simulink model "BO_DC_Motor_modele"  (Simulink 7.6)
settings: Solver=ode15s  StartTime=0.0  StopTime=100  RelTol=1e-3
StopFcn:
  | load BO_pos_vit.mat
  | delete *.mat
  | plot(x(1,:),x(2,:), x(1,:),x(3,:),x(1,:),x(4,:),'*')
  | grid
  | title('Commande en BO de la vitesse linéaire du Moteur DC')
  | gtext('Commande)')
  | gtext('Vitesse linéaire')
  | xlabel('temps')
libraries: fl_lib x13, nesl_utility x4, elec_lib x1

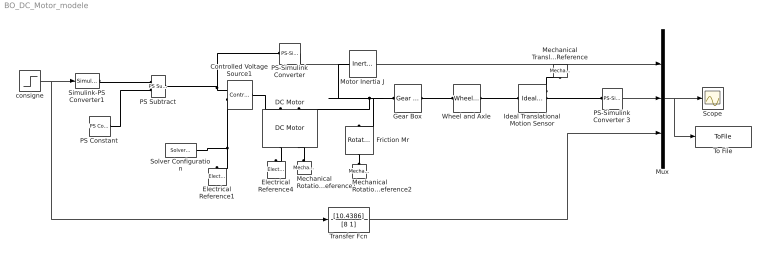
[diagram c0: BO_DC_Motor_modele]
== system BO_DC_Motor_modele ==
  Controlled Voltage Source1 : fl_lib/Electrical/Electrical Sources/Controlled Voltage Source  DialogController=NetworkEngine.DynNeDlgSource  SystemSampleTime=-1  i_Log=off  v_Log=off  LocalVarNames=|current|voltage|power  LocalVarDescs=|Current (A)|Voltage (V)|Power (W)  LocalVarLogging=[0 0 0]
  DC Motor : elec_lib/Actuators & Drivers/Rotational Actuators/DC Motor  DialogController=NetworkEngine.DynNeDlgSource  SystemSampleTime=-1  parameterization=1  Ra=3.9 Ohm  La=1.2e-05 H  emf_or_torque=1  Kv=7.2e-05 V/rpm  Ki=6.876e-04 N*m/A  T_stall=2.4e-04 N*m  w_max=1.91e+04 rpm  w_rated=1.5e+04 rpm  P_rated=0.08 W  V_rated=1.5 V  J=0.01 g*cm^2  lam=1e-08 N*m/(rad/s)  speed0=0 rpm  current_Log=off  voltage_Log=off  power_Log=off  i2r_Log=off  torque_Log=off  speed_Log=off  LocalVarNames=|current|voltage|power|i2r|torque|speed  LocalVarDescs=|Current (A)|Voltage (V)|Power (W)|Electrical losses (W)|Torque (Nm)|Angular speed (rad/s)  LocalVarLogging=[0 0 0 0 0 0]
  Electrical Reference1 : fl_lib/Electrical/Electrical Elements/Electrical Reference  DialogController=NetworkEngine.DynNeDlgSource  SystemSampleTime=-1  i_Log=off  LocalVarNames=|i  LocalVarDescs=|i  LocalVarLogging=[]
  Electrical Reference4 : fl_lib/Electrical/Electrical Elements/Electrical Reference  DialogController=NetworkEngine.DynNeDlgSource  SystemSampleTime=-1  i_Log=off  LocalVarNames=|i  LocalVarDescs=|i  LocalVarLogging=[]
  Friction Mr : fl_lib/Mechanical/Rotational Elements/Rotational Friction  DialogController=NetworkEngine.DynNeDlgSource  SystemSampleTime=-1  brkwy_trq=0.02e-3 N*m  Col_trq=0.02e-3 N*m  visc_coef=0 N*m/(rad/s)  trans_coef=10 s/rad  vel_thr=0.1 rad/s  t_Log=off  w_Log=off  LocalVarNames=|friction_torque|rel_velocity|power  LocalVarDescs=|Friction torque (N*m)|Relative velocity (rad/s)|Power (W)  LocalVarLogging=[0 0 0]
  Gear Box : fl_lib/Mechanical/Mechanisms/Gear Box  DialogController=NetworkEngine.DynNeDlgSource  SystemSampleTime=-1  ratio=5  t_in_Log=off  t_out_Log=off  LocalVarNames=|t_in|t_out  LocalVarDescs=|t_in|t_out  LocalVarLogging=[0 0]
  Ideal Translational Motion Sensor : fl_lib/Mechanical/Mechanical Sensors/Ideal Translational Motion Sensor  DialogController=NetworkEngine.DynNeDlgSource  SystemSampleTime=-1  offset=0 m  v_Log=off  f_Log=off  x_Log=off  LocalVarNames=|v|f|x  LocalVarDescs=|v|f|x  LocalVarLogging=[0 0 0]
  Mechanical Rotational Reference1 : fl_lib/Mechanical/Rotational Elements/Mechanical Rotational Reference  DialogController=NetworkEngine.DynNeDlgSource  SystemSampleTime=-1  t_Log=off  LocalVarNames=|t  LocalVarDescs=|t  LocalVarLogging=[]
  Mechanical Rotational Reference2 : fl_lib/Mechanical/Rotational Elements/Mechanical Rotational Reference  DialogController=NetworkEngine.DynNeDlgSource  SystemSampleTime=-1  t_Log=off  LocalVarNames=|t  LocalVarDescs=|t  LocalVarLogging=[]
  Mechanical Translational Reference : fl_lib/Mechanical/Translational Elements/Mechanical Translational Reference  DialogController=NetworkEngine.DynNeDlgSource  SystemSampleTime=-1  f_Log=off  LocalVarNames=|f  LocalVarDescs=|f  LocalVarLogging=0
  Motor Inertia J : fl_lib/Mechanical/Rotational Elements/Inertia  DialogController=NetworkEngine.DynNeDlgSource  SystemSampleTime=-1  inertia=10 g*cm^2  initial_velocity=0 rad/s  t_Log=off  LocalVarNames=|torque|velocity  LocalVarDescs=|Inertia torque (N*m)|Inertia absolute velocity (rad/s)  LocalVarLogging=[0 0]
  Mux : Mux  Inputs=3
  PS Constant : fl_lib/Physical Signals/Sources/PS Constant  DialogController=NetworkEngine.DynNeDlgSource  SystemSampleTime=-1  constant=0  LocalVarLogging=[]
  PS Subtract : fl_lib/Physical Signals/Functions/PS Subtract  DialogController=NetworkEngine.DynNeDlgSource  SystemSampleTime=-1  LocalVarLogging=[]
  PS-Simulink Converter : nesl_utility/PS-Simulink Converter  DialogController=NetworkEngine.DynNeUtilDlgSource  SystemSampleTime=-1  PhysicalDomain=network_engine_domain  LeftPortType=input  RightPortType=output  SubClassName=ps_output  Unit=1  AffineConversion=off
  PS-Simulink Converter 3 : nesl_utility/PS-Simulink Converter  DialogController=NetworkEngine.DynNeUtilDlgSource  SystemSampleTime=-1  PhysicalDomain=network_engine_domain  LeftPortType=input  RightPortType=output  SubClassName=ps_output  Unit=1  AffineConversion=off
  Scope : Scope
  Simulink-PS Converter1 : nesl_utility/Simulink-PS Converter  DialogController=NetworkEngine.DynNeUtilDlgSource  SystemSampleTime=-1  PhysicalDomain=network_engine_domain  LeftPortType=input  RightPortType=output  SubClassName=ps_input  Unit=1  AffineConversion=off  InputFilterTimeConstant=.001  UdotUserProvided=0
  Solver Configuration : nesl_utility/Solver Configuration  DialogController=NetworkEngine.DynNeUtilDlgSource  SystemSampleTime=-1  PhysicalDomain=network_engine_domain  LeftPortType=input  RightPortType=generic  SubClassName=solver  Accelerate=off  Profile=off  ResidualTolerance=1e-9  MaxNonlinIter=12  MaxModeIter=2  DoFixedCost=off  UseLocalSampling=off  DoDC=off  LinearAlgebra=Full  LocalSolverSampleTime=.001  LocalSolverChoice=NE_BACKWARD_EULER_ADVANCER  UseLocalSolver=off
  To File : ToFile  Filename=BO_pos_vit.mat  MatrixName=x
  Transfer Fcn : TransferFcn  Numerator=[10.4386]  Denominator=[8 1]
  Wheel and Axle : fl_lib/Mechanical/Mechanisms/Wheel and Axle  DialogController=NetworkEngine.DynNeDlgSource  SystemSampleTime=-1  R=0.05 m  or=1  torque_A_Log=off  force_P_Log=off  ang_velocity_Log=off  velocity_Log=off  LocalVarNames=|torque_A|force_P|ang_velocity|velocity  LocalVarDescs=|Axle torque (N*m)|Periphery force (N)|Axle angular velocity (rad/s)|Periphery velocity (m/s)  LocalVarLogging=[0 0 0 0]
  consigne : Step  Time=10  After=0.5  SampleTime=0
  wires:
  Mux/1 -> To File/1, Scope/1
  consigne/1 -> Simulink-PS Converter1/1, Transfer Fcn/1
  PS-Simulink Converter 3/1 -> Mux/2
  PS-Simulink Converter/1 -> Mux/1
  Transfer Fcn/1 -> Mux/3
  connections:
  Ideal Translational Motion Sensor/RConn1 -- Mechanical Translational Reference/LConn1
  Simulink-PS Converter1/RConn1 -- PS Subtract/LConn1
  Mechanical Rotational Reference1/LConn1 -- DC Motor/RConn2
  Gear Box/LConn1 -- Motor Inertia J/LConn1 -- DC Motor/LConn2 -- Friction Mr/LConn1
  Wheel and Axle/LConn1 -- Gear Box/RConn1
  Wheel and Axle/RConn1 -- Ideal Translational Motion Sensor/LConn1
  Friction Mr/RConn1 -- Mechanical Rotational Reference2/LConn1
  DC Motor/RConn1 -- Electrical Reference4/LConn1
  Controlled Voltage Source1/LConn1 -- DC Motor/LConn1
  Controlled Voltage Source1/RConn2 -- Electrical Reference1/LConn1 -- Solver Configuration/RConn1
  PS-Simulink Converter/LConn1 -- PS Subtract/RConn1 -- Controlled Voltage Source1/RConn1
  PS Constant/RConn1 -- PS Subtract/LConn2
  Ideal Translational Motion Sensor/RConn2 -- PS-Simulink Converter 3/LConn1
